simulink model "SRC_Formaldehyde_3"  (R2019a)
settings: Solver=VariableStepAuto  StartTime=0.0  StopTime=tend  RelTol=1e-3
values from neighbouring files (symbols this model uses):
  alpha_MeOH = u(5)    [Bias_calc.m]
  c_MeOH_0 = m_MeOH_sp_0/(m_MeOH_sp_0+m_air_sp_0)    [Mixer_script.m]
  comp_actuator_0 = [z0actuator,comp_w0]    [Compressor_script.m]
  comp_actuator_par = [comp_act_Ga;comp_act_tau;comp_act_zeta]    [Compressor_script.m]
  comp_deltaP = 2.1    [Compressor_script.m]
  comp_p1 = [a0,a1,a2,a3,b0,b1,b2,c0,c1,c2]    [Compressor_script.m]
  comp_p2 = [rho_a, kappa_a, cp_a, R_a, T_amb, d_c]    [Compressor_script.m]
  I_0_compressor = 0.39275    [Compressor_script.m]
  I_0_valve = valve_z0/valve_act_Ga    (= 0.7)    [Valve_script.m]
  Kc_comp = tau_compfotd/(K_compfotd*(tauc_comp+theta_compfotd))    [Compressor_script.m]
  Kc_mtot_MeOH = tau_mtot_MeOH/(K_mtot_MeOH*(tauc_mtot_MeOH+theta_mtot_MeOH))    (= 0.0903815050899)    [Basic_outer_PID_script.m]
  Kc_SRC = abs(Kc_SRC)    [TuningSRC.m]
  Kc_valve = tau_valvefotd/(K_valvefotd*(tauc_valve+theta_valvefotd))    [Valve_script.m]
  KI_comp = Kc_comp/tauI_comp    [Compressor_script.m]
  KI_mtot_MeOH = Kc_mtot_MeOH/tauI_mtot_MeOH    [Basic_outer_PID_script.m]
  KI_SRC = Kc_SRC/tauI_SRC    [TuningSRC.m]
  KI_valve = Kc_valve/tauI_valve    [Valve_script.m]
  m_MeOH_sp_0 = 2940    [Valve_script.m]
  m_MeOH_sp_step = -m_MeOH_sp_0*0.1    [main_VPC_formaldehyde.m]    (also in main_basic_formaldehyde.m; main_basicTPM_formaldehyde.m; main_SRC_formaldehyde.m)
  m_MeOH_sp_step_time = 20    [main_VPC_formaldehyde.m]    (also in main_basic_formaldehyde.m; main_basicTPM_formaldehyde.m; main_SRC_formaldehyde.m)
  m_tot_sp_0 = m_air_sp_0+m_MeOH_sp_0    [main_VPC_formaldehyde.m]    (also in main_basic_formaldehyde.m; main_basicTPM_formaldehyde.m; main_SRC_formaldehyde.m)
  m_tot_sp_step1 = 0*m_tot_sp_0*0.15    [main_VPC_formaldehyde.m]    (also in main_basic_formaldehyde.m; main_basicTPM_formaldehyde.m; main_SRC_formaldehyde.m)
  m_tot_sp_step2 = 1*m_tot_sp_0*0.10    [main_VPC_formaldehyde.m]    (also in main_basic_formaldehyde.m; main_basicTPM_formaldehyde.m; main_SRC_formaldehyde.m)
  m_tot_sp_step3 = 0*(m_tot_sp_step2+m_tot_sp_step1)    [main_VPC_formaldehyde.m]    (also in main_basic_formaldehyde.m = -1*(m_tot_sp_step2+m_tot_sp_step1); main_basicTPM_formaldehyde.m = -1*(m_tot_sp_step2+m_tot_sp_step1); main_SRC_formaldehyde.m = -1*(m_tot_sp_step2+m_tot_sp_step1))
  m_tot_sp_step_t1 = 20    [main_VPC_formaldehyde.m]    (also in main_basic_formaldehyde.m; main_basicTPM_formaldehyde.m; main_SRC_formaldehyde.m)
  m_tot_sp_step_t2 = 30    [main_VPC_formaldehyde.m]    (also in main_basic_formaldehyde.m; main_basicTPM_formaldehyde.m; main_SRC_formaldehyde.m)
  m_tot_sp_step_t3 = 60    [main_VPC_formaldehyde.m]    (also in main_basic_formaldehyde.m = 70; main_basicTPM_formaldehyde.m = 70; main_SRC_formaldehyde.m = 70)
  mair_max = u(2)    [Bias_calc.m]    (also in Compressor_script.m = 25811.62; MeOHmax.m)
  max_MeOH_PI = m_MeOH_max-m_MeOH_sp_0    [Basic_outer_PID_script.m]
  min_MeOH_PI = m_MeOH_min-m_MeOH_sp_0    [Basic_outer_PID_script.m]
  N_cmax = 10048    [Compressor_script.m]
  N_cmin = 7500    [Compressor_script.m]
  p_mix = [MW_MeOH;MW_air;rho_MeOH;rho_a;V_mixer]    [Mixer_script.m]
  PI_comp_max = 0.2    [Compressor_script.m]
  PI_comp_min = -I_0_compressor    (= -0.39275)    [Compressor_script.m]
  type_of_bias = 1    [main_SRC_formaldehyde.m]
  valve_actuator_0 = [valve_z0 valve_w0]    [Valve_script.m]
  valve_actuator_par = [valve_act_Ga;valve_act_tau;valve_act_zeta]    [Valve_script.m]
  valve_Cv = m_MeOH_max/sqrt(valve_delta_p)    [Valve_script.m]
  valve_delta_p = 0.5    [Valve_script.m]
  valve_type = 3    [Valve_script.m]
  x_MeOH_sp_step1 = 1*-0.005    (= -0.005)    [main_VPC_formaldehyde.m]    (also in main_basic_formaldehyde.m; main_basicTPM_formaldehyde.m; main_SRC_formaldehyde.m)
  x_MeOH_sp_step2 = 0*-0.005    (= 0)    [main_VPC_formaldehyde.m]    (also in main_basic_formaldehyde.m; main_basicTPM_formaldehyde.m; main_SRC_formaldehyde.m)
  x_MeOH_sp_step3 = 0*+0.01    (= 0)    [main_VPC_formaldehyde.m]    (also in main_basic_formaldehyde.m; main_basicTPM_formaldehyde.m; main_SRC_formaldehyde.m)
  x_MeOH_sp_step_t1 = 10    [main_VPC_formaldehyde.m]    (also in main_basic_formaldehyde.m; main_basicTPM_formaldehyde.m; main_SRC_formaldehyde.m)
  x_MeOH_sp_step_t2 = 40    [main_VPC_formaldehyde.m]    (also in main_basic_formaldehyde.m; main_basicTPM_formaldehyde.m; main_SRC_formaldehyde.m)
  x_MeOH_sp_step_t3 = 60    [main_VPC_formaldehyde.m]    (also in main_basic_formaldehyde.m = 70; main_basicTPM_formaldehyde.m = 70; main_SRC_formaldehyde.m = 70)
  x_MeOHsp_0 = 0.1    [main_VPC_formaldehyde.m]    (also in main_basic_formaldehyde.m; main_basicTPM_formaldehyde.m; main_SRC_formaldehyde.m)
undefined symbols (not defined in the file or in its folder): actuator, alpha_air, Bias_calc, Bias_par, compressor, deltam_airsp, deltam_MeOH, m_MeOH_bias_constant, m_MeOHbias, mair_bias, mair_min_max, mixerMeOH_O2_dynamic, mixerMeOH_O2_ss, mMeOH_min_max, norm_inverse, normalize, SR_block, v_0, valve, vmaxPI, vminPI
libraries: simulink x4

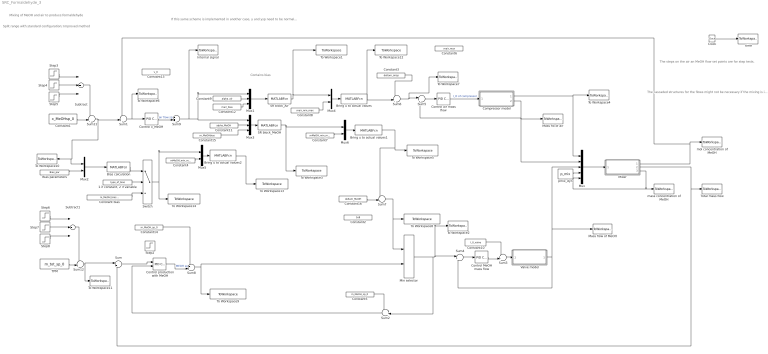
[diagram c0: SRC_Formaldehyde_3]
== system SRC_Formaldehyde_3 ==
  note: Mixing of MeOH and air to produce formaldehyde
  note: The cascaded structures for the flows might not be necessary if the mixing is instantaneous. I just added them to have a general structure. I also added a small residence time in the tank.
  note: The steps on the air an MeOH flow set points are for step tests.
  note: Split range with standard configuration; Improved method
  note: Contains bias
  note: If this same scheme is implemented in another case, y and ysp need to be normalized!!! Here they are not normalized because x_MeOH already goes from 0 to 1
  "1 if constant, 2 if variable" : Constant  Value=type_of_bias
  Bias calculation : MATLABFcn  MATLABFcn=Bias_calc(u)
  Bias parameters : Constant  Value=Bias_par
  Bring u to actual values : MATLABFcn  Description=SR block  MATLABFcn=norm_inverse(u)  OutputDimensions=1
  Bring u to actual values1 : MATLABFcn  Description=SR block  MATLABFcn=norm_inverse(u)  OutputDimensions=1
  Bring u to actual values2 : MATLABFcn  Description=SR block  MATLABFcn=normalize(u)  OutputDimensions=1
  Clock : Clock
  Compressor model : Subsystem
  Constant bias : Constant  Value=m_MeOH_bias_constant
  Constant1 : Constant  Value=x_MeOHsp_0
  Constant10 : Constant  Value=I_0_valve
  Constant11 : Constant  Value=alpha_MeOH
  Constant12 : Constant  Value=mair_bias
  Constant13 : Constant  Value=v_0
  Constant14 : Constant  Value=m_MeOH_sp_0
  Constant15 : Constant  Value=m_MeOHbias
  Constant16 : Constant  Value=deltam_MeOH
  Constant2 : Constant  Value=1e8
  Constant3 : Constant  Value=deltam_airsp
  Constant4 : Constant  Value=mMeOH_min_max
  Constant5 : Constant  Value=m_MeOH_sp_0
  Constant6 : Constant  Value=mair_max
  Constant7 : Constant  Value=mMeOH_min_max
  Constant8 : Constant  Value=mair_min_max
  Constant9 : Constant  Value=alpha_air
  Control MeOH mass flow : simulink/Continuous/PID Controller  Controller=PI  Form=Parallel  TimeDomain=Continuous-time  SampleTime=-1  IntegratorMethod=Forward Euler  FilterMethod=Forward Euler  ControllerParametersSource=internal  P=Kc_valve  I=KI_valve  D=0  UseFilter=on  N=100  TunerSelectOption=Transfer Function Based (PID Tuner App)  InitialConditionSource=internal  InitialConditionForIntegrator=0  InitialConditionForFilter=0  DifferentiatorICPrevScaledInput=0  ExternalReset=none  TrackingMode=off  Kt=1  LimitOutput=on  UpperSaturationLimit=1-I_0_valve  LowerSaturationLimit=-I_0_valve  LinearizeAsGain=on  AntiWindupMode=back-calculation  Kb=1  POutMin=[]  POutMax=[]  IOutMin=[]  IOutMax=[]  DOutMin=[]  DOutMax=[]  NOutMin=[]  NOutMax=[]  SumOutMin=[]  SumOutMax=[]  SaturationOutMin=[]  SaturationOutMax=[]  PParamMin=[]  PParamMax=[]  IParamMin=[]  IParamMax=[]  DParamMin=[]  DParamMax=[]  NParamMin=[]  NParamMax=[]  KbParamMin=[]  KbParamMax=[]  KtParamMin=[]  KtParamMax=[]  KbOutMin=[]  KbOutMax=[]  KtOutMin=[]  KtOutMax=[]  IntegratorOutMin=[]  IntegratorOutMax=[]  FilterOutMin=[]  FilterOutMax=[]  SumI1OutMin=[]  SumI1OutMax=[]  SumI2OutMin=[]  SumI2OutMax=[]  SumI3OutMin=[]  SumI3OutMax=[]  SumI4OutMin=[]  SumI4OutMax=[]  SumDOutMin=[]  SumDOutMax=[]  DifferentiatorOutMin=[]  DifferentiatorOutMax=[]  FilterDiffOutCoefMin=[]  FilterDiffOutCoefMax=[]  ReciprocalOutMin=[]  ReciprocalOutMax=[]  SumDenOutMin=[]  SumDenOutMax=[]  SumNumOutMin=[]  SumNumOutMax=[]  DivideOutMin=[]  DivideOutMax=[]  IntegratorContinuousStateAttributes=''  IntegratorStateMustResolveToSignalObject=off  IntegratorRTWStateStorageClass=Auto  FilterContinuousStateAttributes=''  FilterStateMustResolveToSignalObject=off  FilterRTWStateStorageClass=Auto  ParallelPVariant=InternalParameters  IdealPVariant=Disabled  IVariant=InternalParameters  DVariant=Disabled  IntegratorVariant=Continuous  SatVariant=Enabled  AWVariant=BackCalculation  PCopyVariant=Disabled  TRVariant=Disabled  FdbkBlocksVariant=Forward  IdealPFdbkVariant=Disabled  SatFdbkVariant=Disabled  DerivativeFilterVariant=Disabled  NVariant=Disabled  NCopyVariant=Disabled_SignalSpec  FilterICVariant=Disabled  IntegratorICVariant=InternalICs  ExternalResetVariant=Disabled  TRSumVariant=Passthrough  SumFdbkVariant=Disabled  SumVariant=Sum_PI
  Control air mass flow : simulink/Continuous/PID Controller  Controller=PI  Form=Parallel  TimeDomain=Continuous-time  SampleTime=-1  IntegratorMethod=Forward Euler  FilterMethod=Forward Euler  ControllerParametersSource=internal  P=Kc_comp  I=KI_comp  D=0  UseFilter=on  N=100  TunerSelectOption=Transfer Function Based (PID Tuner App)  InitialConditionSource=internal  InitialConditionForIntegrator=0  InitialConditionForFilter=0  DifferentiatorICPrevScaledInput=0  ExternalReset=none  TrackingMode=off  Kt=1  LimitOutput=on  UpperSaturationLimit=PI_comp_max  LowerSaturationLimit=PI_comp_min  LinearizeAsGain=on  AntiWindupMode=back-calculation  Kb=1  POutMin=[]  POutMax=[]  IOutMin=[]  IOutMax=[]  DOutMin=[]  DOutMax=[]  NOutMin=[]  NOutMax=[]  SumOutMin=[]  SumOutMax=[]  SaturationOutMin=[]  SaturationOutMax=[]  PParamMin=[]  PParamMax=[]  IParamMin=[]  IParamMax=[]  DParamMin=[]  DParamMax=[]  NParamMin=[]  NParamMax=[]  KbParamMin=[]  KbParamMax=[]  KtParamMin=[]  KtParamMax=[]  KbOutMin=[]  KbOutMax=[]  KtOutMin=[]  KtOutMax=[]  IntegratorOutMin=[]  IntegratorOutMax=[]  FilterOutMin=[]  FilterOutMax=[]  SumI1OutMin=[]  SumI1OutMax=[]  SumI2OutMin=[]  SumI2OutMax=[]  SumI3OutMin=[]  SumI3OutMax=[]  SumI4OutMin=[]  SumI4OutMax=[]  SumDOutMin=[]  SumDOutMax=[]  DifferentiatorOutMin=[]  DifferentiatorOutMax=[]  FilterDiffOutCoefMin=[]  FilterDiffOutCoefMax=[]  ReciprocalOutMin=[]  ReciprocalOutMax=[]  SumDenOutMin=[]  SumDenOutMax=[]  SumNumOutMin=[]  SumNumOutMax=[]  DivideOutMin=[]  DivideOutMax=[]  IntegratorContinuousStateAttributes=''  IntegratorStateMustResolveToSignalObject=off  IntegratorRTWStateStorageClass=Auto  FilterContinuousStateAttributes=''  FilterStateMustResolveToSignalObject=off  FilterRTWStateStorageClass=Auto  ParallelPVariant=InternalParameters  IdealPVariant=Disabled  IVariant=InternalParameters  DVariant=Disabled  IntegratorVariant=Continuous  SatVariant=Enabled  AWVariant=BackCalculation  PCopyVariant=Disabled  TRVariant=Disabled  FdbkBlocksVariant=Forward  IdealPFdbkVariant=Disabled  SatFdbkVariant=Disabled  DerivativeFilterVariant=Disabled  NVariant=Disabled  NCopyVariant=Disabled_SignalSpec  FilterICVariant=Disabled  IntegratorICVariant=InternalICs  ExternalResetVariant=Disabled  TRSumVariant=Passthrough  SumFdbkVariant=Disabled  SumVariant=Sum_PI
  Control production with MeOH : simulink/Continuous/PID Controller  Controller=PI  Form=Parallel  TimeDomain=Continuous-time  SampleTime=-1  IntegratorMethod=Forward Euler  FilterMethod=Forward Euler  ControllerParametersSource=internal  P=Kc_mtot_MeOH  I=KI_mtot_MeOH  D=0  UseFilter=on  N=100  TunerSelectOption=Transfer Function Based (PID Tuner App)  InitialConditionSource=internal  InitialConditionForIntegrator=0  InitialConditionForFilter=0  DifferentiatorICPrevScaledInput=0  ExternalReset=none  TrackingMode=on  Kt=1  LimitOutput=on  UpperSaturationLimit=max_MeOH_PI  LowerSaturationLimit=min_MeOH_PI  LinearizeAsGain=on  AntiWindupMode=back-calculation  Kb=1  POutMin=[]  POutMax=[]  IOutMin=[]  IOutMax=[]  DOutMin=[]  DOutMax=[]  NOutMin=[]  NOutMax=[]  SumOutMin=[]  SumOutMax=[]  SaturationOutMin=[]  SaturationOutMax=[]  PParamMin=[]  PParamMax=[]  IParamMin=[]  IParamMax=[]  DParamMin=[]  DParamMax=[]  NParamMin=[]  NParamMax=[]  KbParamMin=[]  KbParamMax=[]  KtParamMin=[]  KtParamMax=[]  KbOutMin=[]  KbOutMax=[]  KtOutMin=[]  KtOutMax=[]  IntegratorOutMin=[]  IntegratorOutMax=[]  FilterOutMin=[]  FilterOutMax=[]  SumI1OutMin=[]  SumI1OutMax=[]  SumI2OutMin=[]  SumI2OutMax=[]  SumI3OutMin=[]  SumI3OutMax=[]  SumI4OutMin=[]  SumI4OutMax=[]  SumDOutMin=[]  SumDOutMax=[]  DifferentiatorOutMin=[]  DifferentiatorOutMax=[]  FilterDiffOutCoefMin=[]  FilterDiffOutCoefMax=[]  ReciprocalOutMin=[]  ReciprocalOutMax=[]  SumDenOutMin=[]  SumDenOutMax=[]  SumNumOutMin=[]  SumNumOutMax=[]  DivideOutMin=[]  DivideOutMax=[]  IntegratorContinuousStateAttributes=''  IntegratorStateMustResolveToSignalObject=off  IntegratorRTWStateStorageClass=Auto  FilterContinuousStateAttributes=''  FilterStateMustResolveToSignalObject=off  FilterRTWStateStorageClass=Auto  ParallelPVariant=InternalParameters  IdealPVariant=Disabled  IVariant=InternalParameters  DVariant=Disabled  IntegratorVariant=Continuous  SatVariant=Enabled  AWVariant=BackCalculation  PCopyVariant=Disabled  TRVariant=Enabled  FdbkBlocksVariant=Forward  IdealPFdbkVariant=Disabled  SatFdbkVariant=Disabled  DerivativeFilterVariant=Disabled  NVariant=Disabled  NCopyVariant=Disabled_SignalSpec  FilterICVariant=Disabled  IntegratorICVariant=InternalICs  ExternalResetVariant=Disabled  TRSumVariant=TrackingMode  SumFdbkVariant=Disabled  SumVariant=Sum_PI
  "Control x_MeOH " : simulink/Continuous/PID Controller  Controller=PI  Form=Parallel  TimeDomain=Continuous-time  SampleTime=-1  IntegratorMethod=Forward Euler  FilterMethod=Forward Euler  ControllerParametersSource=internal  P=Kc_SRC  I=KI_SRC  D=0  UseFilter=on  N=100  TunerSelectOption=Transfer Function Based (PID Tuner App)  InitialConditionSource=internal  InitialConditionForIntegrator=0  InitialConditionForFilter=0  DifferentiatorICPrevScaledInput=0  ExternalReset=none  TrackingMode=off  Kt=1  LimitOutput=on  UpperSaturationLimit=vmaxPI  LowerSaturationLimit=vminPI  LinearizeAsGain=on  AntiWindupMode=back-calculation  Kb=1  POutMin=[]  POutMax=[]  IOutMin=[]  IOutMax=[]  DOutMin=[]  DOutMax=[]  NOutMin=[]  NOutMax=[]  SumOutMin=[]  SumOutMax=[]  SaturationOutMin=[]  SaturationOutMax=[]  PParamMin=[]  PParamMax=[]  IParamMin=[]  IParamMax=[]  DParamMin=[]  DParamMax=[]  NParamMin=[]  NParamMax=[]  KbParamMin=[]  KbParamMax=[]  KtParamMin=[]  KtParamMax=[]  KbOutMin=[]  KbOutMax=[]  KtOutMin=[]  KtOutMax=[]  IntegratorOutMin=[]  IntegratorOutMax=[]  FilterOutMin=[]  FilterOutMax=[]  SumI1OutMin=[]  SumI1OutMax=[]  SumI2OutMin=[]  SumI2OutMax=[]  SumI3OutMin=[]  SumI3OutMax=[]  SumI4OutMin=[]  SumI4OutMax=[]  SumDOutMin=[]  SumDOutMax=[]  DifferentiatorOutMin=[]  DifferentiatorOutMax=[]  FilterDiffOutCoefMin=[]  FilterDiffOutCoefMax=[]  ReciprocalOutMin=[]  ReciprocalOutMax=[]  SumDenOutMin=[]  SumDenOutMax=[]  SumNumOutMin=[]  SumNumOutMax=[]  DivideOutMin=[]  DivideOutMax=[]  IntegratorContinuousStateAttributes=''  IntegratorStateMustResolveToSignalObject=off  IntegratorRTWStateStorageClass=Auto  FilterContinuousStateAttributes=''  FilterStateMustResolveToSignalObject=off  FilterRTWStateStorageClass=Auto  ParallelPVariant=InternalParameters  IdealPVariant=Disabled  IVariant=InternalParameters  DVariant=Disabled  IntegratorVariant=Continuous  SatVariant=Enabled  AWVariant=BackCalculation  PCopyVariant=Disabled  TRVariant=Disabled  FdbkBlocksVariant=Forward  IdealPFdbkVariant=Disabled  SatFdbkVariant=Disabled  DerivativeFilterVariant=Disabled  NVariant=Disabled  NCopyVariant=Disabled_SignalSpec  FilterICVariant=Disabled  IntegratorICVariant=InternalICs  ExternalResetVariant=Disabled  TRSumVariant=Passthrough  SumFdbkVariant=Disabled  SumVariant=Sum_PI
  Internal signal : ToWorkspace  VariableName=v  SampleTime=-1
  Mass flo of air : ToWorkspace  VariableName=m_air  SampleTime=-1
  Mass flow of MeOH : ToWorkspace  VariableName=m_MeOH  SampleTime=-1
  Min selector : MinMax  Inputs=2
  Mixer : Subsystem
  Mux : Mux  Inputs=5
  Mux1 : Mux  Inputs=3
  Mux{2,4..6} (4 alike) : Mux  Inputs=2
  Mux3 : Mux  Inputs=3
  SR block_Air : MATLABFcn  Description=SR block  MATLABFcn=SR_block(u)  OutputDimensions=1
  SR block_MeOH : MATLABFcn  Description=SR block  MATLABFcn=SR_block(u)  OutputDimensions=1
  Step2 : Step  Time=m_MeOH_sp_step_time  After=m_MeOH_sp_step  SampleTime=0
  Step3 : Step  Time=x_MeOH_sp_step_t1  After=x_MeOH_sp_step1  SampleTime=0
  Step4 : Step  Time=x_MeOH_sp_step_t2  After=x_MeOH_sp_step2  SampleTime=0
  Step5 : Step  Time=x_MeOH_sp_step_t3  After=x_MeOH_sp_step3  SampleTime=0
  Step6 : Step  Time=m_tot_sp_step_t1  After=m_tot_sp_step1  SampleTime=0
  Step7 : Step  Time=m_tot_sp_step_t2  After=m_tot_sp_step2  SampleTime=0
  Step8 : Step  Time=m_tot_sp_step_t3  After=m_tot_sp_step3  SampleTime=0
  Subtract : Sum  Inputs=+++
  Subtract1 : Sum  Inputs=+++
  Sum : Sum  Inputs=|+-
  Sum1 : Sum  Inputs=-+|
  Sum{3,8..9,11..12} (5 alike) : Sum  Inputs=++|
  Sum2 : Sum  Inputs=-+|
  Sum4 : Sum  Inputs=|+-
  Sum5 : Sum  Inputs=|+-
  Sum6 : Sum  Inputs=-+|
  Sum7 : Sum  Inputs=+-|
  Switch : Switch  Criteria=u2 > Threshold  Threshold=1
  TPM : Constant  Value=m_tot_sp_0
  To Workspace1 : ToWorkspace  VariableName=u_air_scaled  SampleTime=-1
  To Workspace10 : ToWorkspace  VariableName=x_MeOHsp  SampleTime=-1
  To Workspace11 : ToWorkspace  VariableName=m_tot_sp  SampleTime=-1
  To Workspace12 : ToWorkspace  VariableName=u_air  SampleTime=-1
  To Workspace13 : ToWorkspace  VariableName=bias_MeOH_norm  SampleTime=-1
  To Workspace14 : ToWorkspace  VariableName=bias_MeOH  SampleTime=-1
  To Workspace2 : ToWorkspace  VariableName=m_MEOH_sp  SampleTime=-1
  To Workspace3 : ToWorkspace  VariableName=u_MeOH_scaled  SampleTime=-1
  To Workspace4 : ToWorkspace  VariableName=Q_air  SampleTime=-1
  To Workspace5 : ToWorkspace  VariableName=u_MeOH  SampleTime=-1
  To Workspace6 : ToWorkspace  VariableName=x_MeOH_error  SampleTime=-1
  To Workspace7 : ToWorkspace  VariableName=m_air_sp  SampleTime=-1
  To Workspace8 : ToWorkspace  VariableName=m_MEOH_sp_SR  SampleTime=-1
  To Workspace9 : ToWorkspace  VariableName=m_MeOH_sp_m_tot  SampleTime=-1
  Total mass flow : ToWorkspace  VariableName=m_tot  SampleTime=-1
  Valve model : Subsystem
  mass concentration of MeOH : ToWorkspace  VariableName=c_MeOH  SampleTime=-1
  mol concentration of MeOH : ToWorkspace  VariableName=x_MeOH  SampleTime=-1
  pmix_dyn : Constant  Value=p_mix
  time : ToWorkspace  VariableName=t  SampleTime=-1
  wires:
  Valve model/1(m_MeOH) -> Mass flow of MeOH/1, Mux/3, Sum4/2
  Clock/1 -> time/1
  Compressor model/2(m_air) -> Sum5/2, Mux/2, Mass flo of air/1
  Compressor model/1(Q_air) -> Mux/1, To Workspace4/1
  Control MeOH mass flow/1 -> Sum3/2
  Constant10/1 -> Sum3/1
  Sum4/1 -> Control MeOH mass flow/1
  Mixer/2(m_tot) -> Total mass flow/1, Sum/2
  Mixer/1(x_MeOH) -> Sum1/1, mol concentration of MeOH/1
  pmix_dyn/1 -> Mux/4
  Constant14/1 -> Sum8/1
  Constant1/1 -> Sum11/2
  Sum11/1 -> Sum1/2, To Workspace10/1, Mux2/1
  Step3/1 -> Subtract/1
  Step4/1 -> Subtract/2
  Step5/1 -> Subtract/3
  TPM/1 -> Sum12/2
  Sum12/1 -> To Workspace11/1, Sum/1
  Step6/1 -> Subtract1/1
  Step7/1 -> Subtract1/2
  Step8/1 -> Subtract1/3
  Subtract1/1 -> Sum12/1
  Control air mass flow/1 -> Compressor model/1(I_blower)  "I_O of compressor"
  Sum5/1 -> Control air mass flow/1
  Mux/1 -> Mixer/1(Mix_par)
  Mixer/3(c_MeOH) -> Mux/5, mass concentration of MeOH/1
  Sum3/1 -> Valve model/1(I_valve)
  Sum/1 -> Control production with MeOH/1
  Sum8/1 -> To Workspace9/1, Min selector/2
  Min selector/1 -> Sum2/2, To Workspace2/1, Sum4/1
  Constant bias/1 -> Switch/3
  "1 if constant, 2 if variable"/1 -> Switch/2
  Bias calculation/1 -> Switch/1
  Mux2/1 -> Bias calculation/1
  Bias parameters/1 -> Mux2/2
  Bring u to actual values/1 -> To Workspace12/1, Sum6/2
  Subtract/1 -> Sum11/1
  Constant5/1 -> Sum2/1
  Sum2/1 -> Control production with MeOH/2
  Sum1/1 -> To Workspace6/1, "Control x_MeOH "/1
  Bring u to actual values1/1 -> Sum7/1, To Workspace5/1
  Mux1/1 -> SR block_Air/1
  Mux3/1 -> SR block_MeOH/1
  SR block_Air/1 -> Mux4/1, To Workspace1/1
  SR block_MeOH/1 -> To Workspace3/1, Mux6/1
  Mux4/1 -> Bring u to actual values/1
  Mux6/1 -> Bring u to actual values1/1
  Mux5/1 -> Bring u to actual values2/1
  Bring u to actual values2/1 -> To Workspace13/1
  Constant4/1 -> Mux5/2
  Constant7/1 -> Mux6/2
  Constant8/1 -> Mux4/2
  Constant9/1 -> Mux1/2
  Constant11/1 -> Mux3/2
  Constant12/1 -> Mux1/3
  Sum7/1 -> Min selector/1, To Workspace8/1
  Switch/1 -> Mux5/1, To Workspace14/1
  Sum6/1 -> Sum5/1, To Workspace7/1
  Constant16/1 -> Sum7/2
  Constant15/1 -> Mux3/3
  "Control x_MeOH "/1 -> Sum9/2  "air flow sp"
  Sum9/1 -> Internal signal/1, Mux1/1, Mux3/1
  Constant3/1 -> Sum6/1
  Control production with MeOH/1 -> Sum8/2  "MEOH sp"

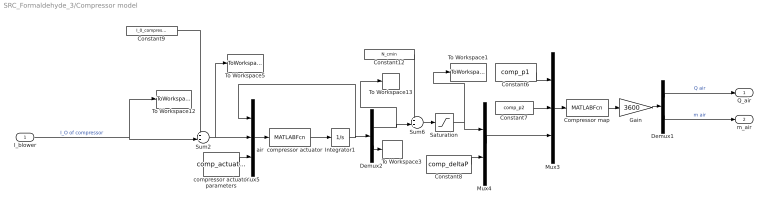
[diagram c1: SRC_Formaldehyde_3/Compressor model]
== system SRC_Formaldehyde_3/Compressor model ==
  I_blower : Inport
  Compressor map : MATLABFcn  MATLABFcn=compressor(u(1:10),u(11:16),u(17:18))  OutputDimensions=2
  Constant12 : Constant  Value=N_cmin
  Constant6 : Constant  Value=comp_p1
  Constant7 : Constant  Value=comp_p2
  Constant8 : Constant  Value=comp_deltaP
  Constant9 : Constant  Value=I_0_compressor
  Demux1 : Demux  Outputs=2
  Demux2 : Demux  Outputs=2
  Gain : Gain  Gain=3600
  Integrator1 : Integrator  InitialCondition=comp_actuator_0
  Mux3 : Mux  Inputs=3
  Mux4 : Mux  Inputs=2
  Mux5 : Mux  Inputs=3
  Saturation : Saturate  UpperLimit=N_cmax  LowerLimit=N_cmin
  Sum2 : Sum  Inputs=++|
  Sum6 : Sum  Inputs=++|
  To Workspace1 : ToWorkspace  VariableName=comp_rpm  SampleTime=-1
  To Workspace12 : ToWorkspace  VariableName=I_air0  SampleTime=-1
  To Workspace13 : ToWorkspace  VariableName=Nc_act1  SampleTime=-1
  To Workspace3 : ToWorkspace  VariableName=wcomp  SampleTime=-1
  To Workspace5 : ToWorkspace  VariableName=I_air  SampleTime=-1
  air  compressor actuator : MATLABFcn  MATLABFcn=actuator(u(1:2),u(3),u(4:6))  OutputDimensions=2
  compressor actuator parameters : Constant  Value=comp_actuator_par
  Q_air : Outport
  m_air : Outport  Port=2
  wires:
  I_blower/1 -> To Workspace12/1, Sum2/2  "I_O of compressor"
  Constant9/1 -> Sum2/1
  Sum6/1 -> Saturation/1
  Constant12/1 -> Sum6/1
  Constant6/1 -> Mux3/1
  Mux5/1 -> air  compressor actuator/1
  Sum2/1 -> To Workspace5/1, Mux5/2
  Integrator1/1 -> Demux2/1, Mux5/1
  Demux2/1 -> To Workspace13/1, Sum6/2
  air  compressor actuator/1 -> Integrator1/1
  Constant8/1 -> Mux4/2
  Demux2/2 -> To Workspace3/1
  Demux1/1 -> Q_air/1  "Q air"
  Mux3/1 -> Compressor map/1
  Constant7/1 -> Mux3/2
  Mux4/1 -> Mux3/3
  Saturation/1 -> To Workspace1/1, Mux4/1
  Compressor map/1 -> Gain/1
  Gain/1 -> Demux1/1
  Demux1/2 -> m_air/1  "m air"
  compressor actuator parameters/1 -> Mux5/3

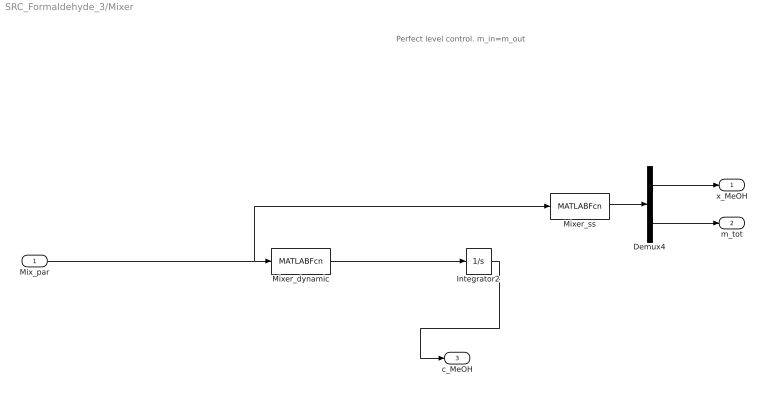
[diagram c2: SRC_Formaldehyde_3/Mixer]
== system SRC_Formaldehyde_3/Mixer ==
  note: Perfect level control. m_in=m_out
  Mix_par : Inport
  Demux4 : Demux  Outputs=2
  Integrator2 : Integrator  InitialCondition=c_MeOH_0
  Mixer_dynamic : MATLABFcn  MATLABFcn=mixerMeOH_O2_dynamic(u(1:3),u(4:8),u(9))  OutputDimensions=1
  Mixer_ss : MATLABFcn  MATLABFcn=mixerMeOH_O2_ss(u(1:3),u(4:8),u(9))  OutputDimensions=2
  x_MeOH : Outport
  m_tot : Outport  Port=2
  c_MeOH : Outport  Port=3
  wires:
  Integrator2/1 -> c_MeOH/1
  Mix_par/1 -> Mixer_ss/1, Mixer_dynamic/1
  Mixer_dynamic/1 -> Integrator2/1
  Mixer_ss/1 -> Demux4/1
  Demux4/1 -> x_MeOH/1
  Demux4/2 -> m_tot/1

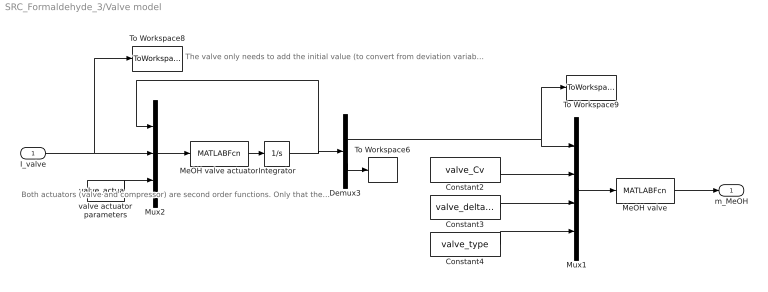
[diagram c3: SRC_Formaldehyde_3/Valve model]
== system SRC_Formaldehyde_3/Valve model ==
  note: The valve only needs to add the initial value (to convert from deviation variables to actual variables "once" before the actuator. The compressor also needs it before the actuator because the range does not start in 0. (Maybe there is a better way to do this).
  note: Both actuators (valve and compressor) are second order functions. Only that the time constants and the damping factors are different.
  I_valve : Inport
  Constant2 : Constant  Value=valve_Cv
  Constant3 : Constant  Value=valve_delta_p
  Constant4 : Constant  Value=valve_type
  Demux3 : Demux  Outputs=2
  Integrator : Integrator  InitialCondition=valve_actuator_0
  MeOH valve : MATLABFcn  MATLABFcn=valve(u)  OutputDimensions=1
  MeOH valve actuator : MATLABFcn  MATLABFcn=actuator(u(1:2),u(3),u(4:6))  OutputDimensions=2
  Mux1 : Mux
  Mux2 : Mux  Inputs=3
  To Workspace6 : ToWorkspace  VariableName=wvalve  SampleTime=-1
  To Workspace8 : ToWorkspace  VariableName=I_MeOH  SampleTime=-1
  To Workspace9 : ToWorkspace  VariableName=z_MeOH  SampleTime=-1
  valve actuator parameters : Constant  Value=valve_actuator_par
  m_MeOH : Outport
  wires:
  Demux3/2 -> To Workspace6/1
  Demux3/1 -> To Workspace9/1, Mux1/1
  MeOH valve actuator/1 -> Integrator/1
  Integrator/1 -> Demux3/1, Mux2/1
  Constant4/1 -> Mux1/4
  Constant3/1 -> Mux1/3
  I_valve/1 -> To Workspace8/1, Mux2/2
  Constant2/1 -> Mux1/2
  Mux2/1 -> MeOH valve actuator/1
  Mux1/1 -> MeOH valve/1
  valve actuator parameters/1 -> Mux2/3
  MeOH valve/1 -> m_MeOH/1
